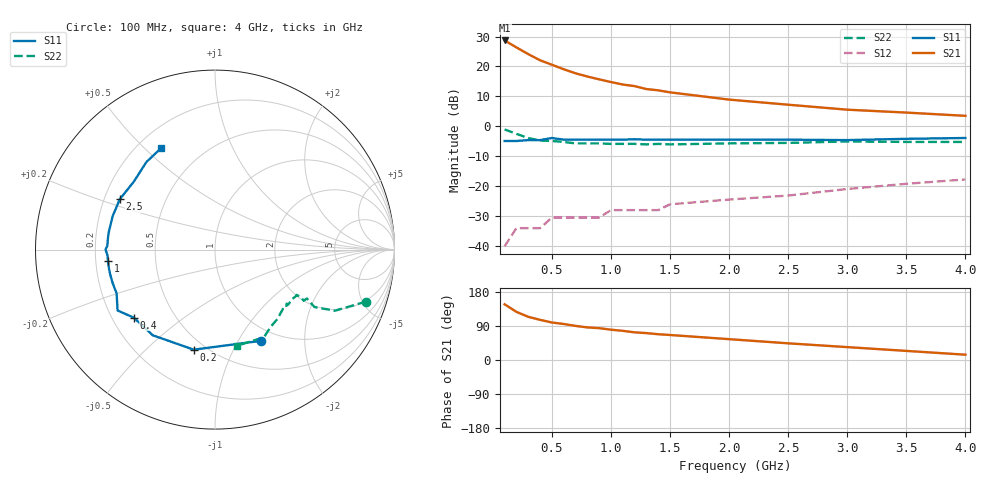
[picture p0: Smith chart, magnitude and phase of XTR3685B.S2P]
!  HXTR-3685 Typical S-Parameters
!  (Vce = 10 V, Ic = 15 mA)
# ghz s ma r 50
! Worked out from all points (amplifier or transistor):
!   20 points, 100 MHz to 4 GHz, reference 50 ohm
!   highest |S21| = 28.7 dB at 100 MHz (marker M1)
!   |S21| within 3 dB of that: start of sweep to 230.1 MHz
!   unconditionally stable (mu >= 1): 827 MHz to 942.5 MHz; 1.12 GHz to 3.25 GHz
!   at 400 MHz: K = 0.72, MSG = 28.0 dB, |S12| = -34.0 dB
!   at 1.1 GHz: K = 0.99, MSG = 21.0 dB, |S12| = -28.0 dB
!   at 4 GHz: K = 0.85, MSG = 10.6 dB, |S12| = -17.7 dB
!   S11 on the Smith chart (normalised r, x): 100 MHz: 0.84, -1.26; 200 MHz: 0.43, -0.71; 400 MHz: 0.29, -0.34; 1 GHz: 0.25, -0.05; 2.5 GHz: 0.26, +0.23; 4 GHz: 0.29, +0.56
0.1  0.57 -63.0  27.2 147.0  0.01 65.0  0.89 -19.0
0.2  0.57 -102.0  20.8 127.0  0.02 52.0  0.75 -27.0
0.3  0.59 -126.0  16.1 114.0  0.02 46.0  0.64 -30.0
0.4  0.59 -140.0  12.7 106.0  0.02 45.0  0.58 -28.0
0.5  0.64 -148.0  10.7 99.0  0.03 46.0  0.57 -30.0
0.6  0.6 -156.0  9 95.0  0.03 47.0  0.55 -29.0
0.7  0.6 -162.0  7.7 90.0  0.03 48.0  0.52 -29.0
0.8  0.6 -167.0  6.8 86.0  0.03 49.0  0.52 -30.0
0.9  0.6 -170.0  6.1 84.0  0.03 51.0  0.52 -30.0
1  0.6 -174.0  5.5 80.0  0.04 53.0  0.51 -33.0
1.1  0.6 -177.0  5 77.0  0.04 54.0  0.51 -34.0
1.2  0.61 180.0  4.7 73.0  0.04 55.0  0.51 -37.0
1.3  0.6 178.0  4.2 71.0  0.04 56.0  0.5 -37.0
1.4  0.6 175.0  4 68.0  0.04 57.0  0.51 -39.0
1.5  0.6 171.0  3.7 66.0  0.05 58.0  0.5 -40.0
2  0.6 162.0  2.8 55.0  0.06 61.0  0.52 -48.0
2.5  0.6 152.0  2.3 44.0  0.07 62.0  0.53 -54.0
3  0.59 140.0  1.9 34.0  0.09 62.0  0.56 -61.0
3.5  0.62 128.0  1.7 24.0  0.11 61.0  0.55 -67.0
4  0.64 118.0  1.5 14.0  0.13 58.0  0.55 -77.0
